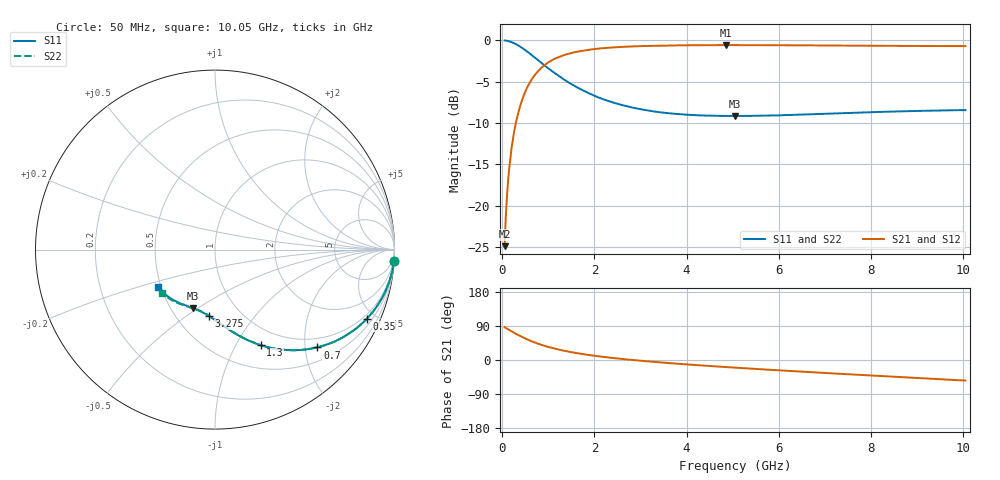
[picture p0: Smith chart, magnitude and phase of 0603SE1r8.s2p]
! AVX Thin Film Operation		Date: August 2001
! Description: Accu-P® Series, Thin Film, SMD, RF Capacitor
! Part Number: 06035J1R8ABT
! 50 MHz  -  10.05 GHz
! Serial Measurements
# mhz S db R 50
!	S11		S21		S12		S22
!	dB	Phase	dB	Phase	dB	Phase	dB	Phase
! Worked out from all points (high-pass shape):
!   401 points, 50 MHz to 10.05 GHz, reference 50 ohm
!   highest |S21| = -0.58 dB at 4.85 GHz (marker M1); lowest = -24.9 dB at 50 MHz (marker M2)
!   |S21| within 3 dB of the highest: 802.6 MHz to end of sweep
!   lowest |S11| = -9.2 dB at 5.05 GHz (marker M3), VSWR 2.07, Z = 32 - j23.7 ohm
!   |S11| at or under -10 dB: nowhere
!   |S22| runs from -9.1 to 0.0 dB; largest |S21 - S12| = 0
!   S11 on the Smith chart (normalised r, x): 50 MHz: 1, -31; 350 MHz: 0.79, -4.49; 700 MHz: 0.78, -2.27; 1.3 GHz: 0.78, -1.27; 3.275 GHz: 0.72, -0.62; 10.05 GHz: 0.48, -0.23
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50  -0.01 -3.7  -24.90 86.3  -24.90 86.3  -0.01 -3.7
75  -0.03 -5.5  -21.41 84.5  -21.41 84.5  -0.03 -5.5
125  -0.09 -9.1  -17.02 80.9  -17.02 80.9  -0.09 -9.1
175  -0.17 -12.6  -14.25 77.4  -14.25 77.4  -0.17 -12.6
250  -0.34 -17.9  -11.28 72.1  -11.28 72.1  -0.34 -17.9
350  -0.63 -24.4  -8.69 65.5  -8.69 65.5  -0.63 -24.4
500  -1.20 -33.4  -6.19 56.6  -6.19 56.6  -1.20 -33.4
700  -2.06 -43.7  -4.24 46.3  -4.24 46.3  -2.06 -43.7
975  -3.28 -54.7  -2.76 35.3  -2.76 35.3  -3.28 -54.7
1125  -3.89 -59.5  -2.28 30.4  -2.28 30.4  -3.89 -59.5
1300  -4.59 -64.5  -1.86 25.5  -1.86 25.5  -4.59 -64.5
1500  -5.29 -69.3  -1.53 20.7  -1.53 20.7  -5.29 -69.2
1725  -5.98 -73.9  -1.27 16.1  -1.27 16.1  -5.98 -73.8
2050  -6.83 -79.7  -1.02 10.4  -1.02 10.4  -6.82 -79.4
2375  -7.47 -84.5  -0.86 5.6  -0.86 5.6  -7.47 -84.1
3275  -8.59 -95.0  -0.66 -4.8  -0.66 -4.8  -8.59 -94.3
3400  -8.68 -96.3  -0.64 -6.1  -0.64 -6.1  -8.67 -95.5
4850  -9.15 -109.6  -0.58 -18.6  -0.58 -18.6  -9.14 -107.6
5050  -9.15 -111.0  -0.58 -20.2  -0.58 -20.2  -9.14 -109.0
6725  -8.94 -123.0  -0.61 -32.3  -0.61 -32.3  -8.92 -121.0
8400  -8.63 -135.2  -0.67 -43.6  -0.67 -43.6  -8.60 -131.1
10050  -8.44 -146.6  -0.70 -54.1  -0.70 -54.1  -8.41 -140.8
